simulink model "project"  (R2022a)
settings: Solver=ode45  StartTime=0.0  StopTime=100  RelTol=1e-3  EnableMultiTasking=on
libraries: simulink x2

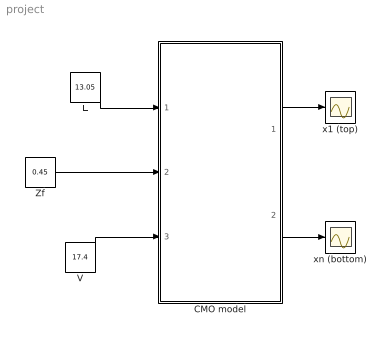
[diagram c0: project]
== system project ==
  CMO model : Subsystem
  L : Constant  Value=13.05
  V : Constant  Value=17.4
  Zf : Constant  Value=0.45
  x1 (top) : Scope
  xn (bottom) : Scope
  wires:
  L/1 -> CMO model/1(In1)
  CMO model/1(Out1) -> x1 (top)/1
  V/1 -> CMO model/3(In3)
  Zf/1 -> CMO model/2(In2)
  CMO model/2(Out3) -> xn (bottom)/1

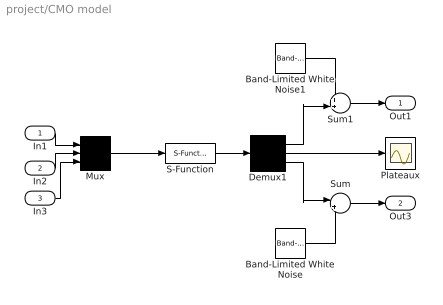
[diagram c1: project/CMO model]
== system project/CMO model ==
  In1 : Inport
  In2 : Inport  Port=2
  In3 : Inport  Port=3
  Band-Limited White Noise : simulink/Sources/Band-Limited White Noise  Cov=[0.0001]  Ts=1  seed=[23341]
  Band-Limited White Noise1 : simulink/Sources/Band-Limited White Noise  Cov=[0.0001]  Ts=1  seed=[23341]
  Demux1 : Demux  Outputs=[1,11,1]
  Mux : Mux  Inputs=3
  Plateaux : Scope
  S-Function : S-Function  FunctionName=CMO_model  SFunctionDeploymentMode=off  EnableBusSupport=off
  Sum : Sum  Inputs=|++
  Sum1 : Sum  Inputs=++|
  Out1 : Outport  InitialOutput=0  VectorParamsAs1DForOutWhenUnconnected=off
  Out3 : Outport  Port=2  VectorParamsAs1DForOutWhenUnconnected=off
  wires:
  In3/1 -> Mux/3
  Demux1/2 -> Plateaux/1
  S-Function/1 -> Demux1/1
  In2/1 -> Mux/2
  In1/1 -> Mux/1
  Mux/1 -> S-Function/1
  Sum/1 -> Out3/1
  Demux1/3 -> Sum/1
  Band-Limited White Noise/1 -> Sum/2
  Sum1/1 -> Out1/1
  Demux1/1 -> Sum1/2
  Band-Limited White Noise1/1 -> Sum1/1
